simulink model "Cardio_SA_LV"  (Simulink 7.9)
settings: Solver=ode1  StartTime=0.0  StopTime=16*T  FixedStep=dt  MinStep=.001  RelTol=1e-3
PreLoadFcn:
  | %Time parameters
  | T = 0.0125;   %Duration of heartbeat (minutes)
  | Ts = 0.0050;   %Duration of systole   (minutes)
  | Stroke_volume = 70e-3;
  | Tmax = 0.0020;  %Time at which flow is max (minutes)
  | Qmax= Stroke_volume/(0.5*Ts);    %Max flow through aortic valve (liters/minute)
  | dt = .00005*T;
  | %This choice implies 20,000 timesteps per cardiac cycle
  | 
  | %Compliance and resistance parameters. Note that valve resistances are not
  | %supposed to be realistic, just small enough to be negligible
  | Csa = .00175; %Systemic arterial compliance (liters/(mmHg))
  | Rs = 17.86; %Systemic resistance (mmHg/(liters/minute))
  | Rmi = .01; %mitral valve resistance (mmHg/(liters/minute))
  | RAo = .01; %Aortic valve resistance (mmHg/(liters/minute))
  | 
  | Vlvd = .027; %Left ventricular volume when PLV = 0 (liters)
  | Vsad = .825; %Systemic arterial volume when Psa = 0 (liters)
  | Pla = 5; %Left atrial pressure (mmHg)
  | 
  | %Parameters for Clv(t)
  | CLVD = .0146; %Max (diastolic) value of CLV (liters/mmHg)
  | CLVS = .00003; %Min (systolic) value of CLV (liters/mmHg)
  | tauS = .0025; %CLV time constant during systole (minutes)
  | tauD = .001; %CLV time constant during diastole (minutes)
  | 
  | %Initialization parameters
  | Plvi = 5; %initial value of PLV (mmHg)
  | Psai = 80; %initial value of Psa (mmHg)
  | 
  | %Don't forget to plot VSA vs. PSA and VLV vs. PLV!!!!!!! The values have
  | %been exported into the matlab workspace so you can plot them yourself!

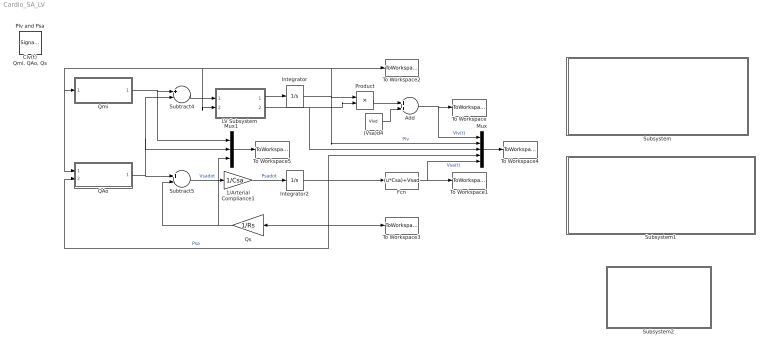
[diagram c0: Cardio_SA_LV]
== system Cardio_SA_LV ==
  (Vsa)d4 : Constant  Value=Vlvd
  1/Arterial Compliance1 : Gain  Gain=1/Csa
  Add : Sum
  Fcn : Fcn  Expr=(u*Csa)+Vsad
  Integrator : Integrator  InitialCondition=Plvi
  Integrator2 : Integrator  InitialCondition=Psai
  LV Subsystem : Subsystem
  Mux : Mux  Inputs=5
  Mux1 : Mux  Inputs=3
  Product : Product
  QAo : Subsystem
  Qmi : Subsystem
  Qs : Gain  Gain=1/Rs
  Subsystem : Subsystem
  Subsystem1 : Subsystem
  Subsystem2 : Subsystem
  Subtract4 : Sum  Inputs=+-
  Subtract5 : Sum  Inputs=+-
  To Workspace : ToWorkspace  VariableName=VLV  SampleTime=-1
  To Workspace1 : ToWorkspace  VariableName=VSA  SampleTime=-1
  To Workspace2 : ToWorkspace  VariableName=PLV  SampleTime=-1
  To Workspace3 : ToWorkspace  VariableName=PSA  SampleTime=-1
  To Workspace4 : ToWorkspace  VariableName=PVClv  SampleTime=-1  SaveFormat=Structure With Time
  To Workspace5 : ToWorkspace  VariableName=BloodFlows  SampleTime=-1  SaveFormat=Structure With Time
  Clv(t) : SignalViewerScope  IOType=viewer  RefreshTime=0.035000
  Plv and Psa : SignalViewerScope  IOType=viewer  RefreshTime=0.035000
  "Qmi, QAo, Qs" : SignalViewerScope  IOType=viewer  RefreshTime=0.035000
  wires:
  Fcn/1 -> To Workspace1/1, Mux/5  "Vsa(t)"
  Subtract5/1 -> 1/Arterial Compliance1/1  "Vsadot"
  1/Arterial Compliance1/1 -> Integrator2/1  "Psadot"
  Integrator2/1 -> Fcn/1, To Workspace3/1, Qs/1, QAo/2(Psa), Mux/4  "Psa"
  Qs/1 -> Subtract5/2, Mux1/3
  QAo/1(Qao) -> Subtract5/1, Subtract4/2, Mux1/2
  Qmi/1(Qmi) -> Subtract4/1, Mux1/1
  Product/1 -> Add/1
  (Vsa)d4/1 -> Add/2
  Add/1 -> To Workspace/1, Mux/1  "Vlv(t)"
  Subtract4/1 -> LV Subsystem/1(Vlddot)
  LV Subsystem/1(Plvdot) -> Integrator/1
  Integrator/1 -> Product/1, To Workspace2/1, LV Subsystem/2(Plv), Qmi/1(Plv), QAo/1(Plv), Mux/2  "Plv"
  LV Subsystem/2(Clv) -> Product/2, Mux/3
  Mux/1 -> To Workspace4/1
  Mux1/1 -> To Workspace5/1

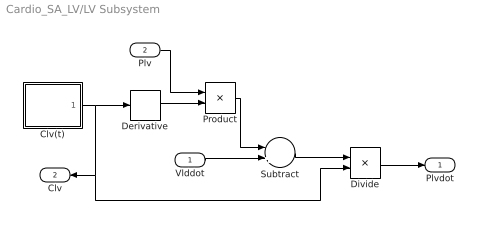
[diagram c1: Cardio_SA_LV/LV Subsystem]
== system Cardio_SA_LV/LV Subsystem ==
  Vlddot : Inport
  Plv : Inport  Port=2
  Clv(t) : Subsystem
  Derivative : Derivative
  Divide : Product  Inputs=*/
  Product : Product
  Subtract : Sum  Inputs=-+
  Plvdot : Outport
  Clv : Outport  Port=2
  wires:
  Clv(t)/1(Clv) -> Derivative/1, Clv/1, Divide/2
  Derivative/1 -> Product/2
  Plv/1 -> Product/1
  Product/1 -> Subtract/1
  Vlddot/1 -> Subtract/2
  Subtract/1 -> Divide/1
  Divide/1 -> Plvdot/1

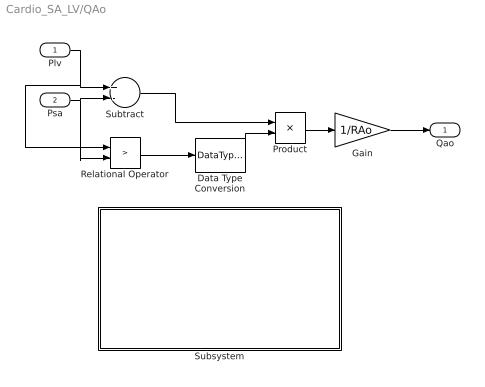
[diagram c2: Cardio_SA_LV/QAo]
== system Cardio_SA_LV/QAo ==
  Plv : Inport
  Psa : Inport  Port=2
  Data Type Conversion : DataTypeConversion  OutDataTypeStr=double
  Gain : Gain  Gain=1/RAo
  Product : Product
  Relational Operator : RelationalOperator  Operator=>  OutDataTypeStr=boolean
  Subsystem : Subsystem
  Subtract : Sum  Inputs=+-
  Qao : Outport
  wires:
  Plv/1 -> Subtract/1, Relational Operator/1
  Subtract/1 -> Product/1
  Product/1 -> Gain/1
  Gain/1 -> Qao/1
  Psa/1 -> Subtract/2, Relational Operator/2
  Data Type Conversion/1 -> Product/2
  Relational Operator/1 -> Data Type Conversion/1

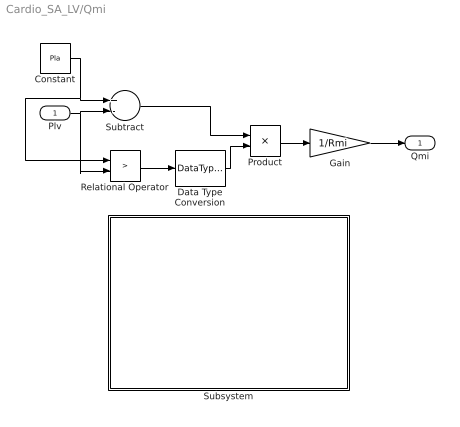
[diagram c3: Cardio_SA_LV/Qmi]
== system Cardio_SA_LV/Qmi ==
  Plv : Inport
  Constant : Constant  Value=Pla
  Data Type Conversion : DataTypeConversion  OutDataTypeStr=double
  Gain : Gain  Gain=1/Rmi
  Product : Product
  Relational Operator : RelationalOperator  Operator=>  OutDataTypeStr=boolean
  Subsystem : Subsystem
  Subtract : Sum  Inputs=+-
  Qmi : Outport
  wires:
  Constant/1 -> Relational Operator/1, Subtract/1
  Subtract/1 -> Product/1
  Product/1 -> Gain/1
  Gain/1 -> Qmi/1
  Plv/1 -> Relational Operator/2, Subtract/2
  Data Type Conversion/1 -> Product/2
  Relational Operator/1 -> Data Type Conversion/1

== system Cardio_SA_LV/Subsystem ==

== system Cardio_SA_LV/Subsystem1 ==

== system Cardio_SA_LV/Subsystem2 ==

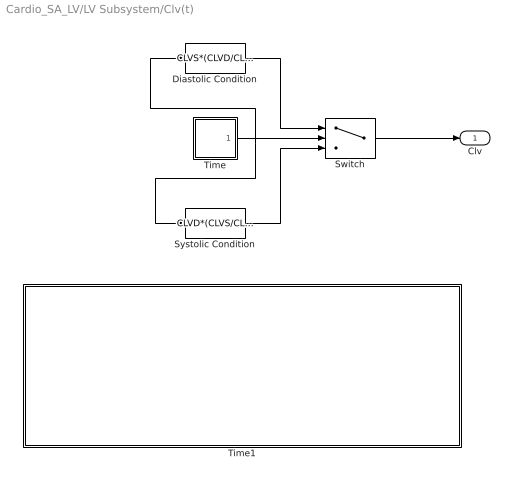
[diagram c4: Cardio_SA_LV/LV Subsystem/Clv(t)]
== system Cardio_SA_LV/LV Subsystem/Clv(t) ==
  Diastolic Condition : Fcn  Expr=CLVS*(CLVD/CLVS)^((1-exp(-(u-Ts)/tauD))/(1-exp(-(T-Ts)/tauD)))
  Switch : Switch  Criteria=u2 > Threshold  Threshold=Ts
  Systolic Condition : Fcn  Expr=CLVD*(CLVS/CLVD)^((1-exp(-u/tauS))/(1-exp(-Ts/tauS)))
  Time : Subsystem
  Time1 : Subsystem
  Clv : Outport
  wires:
  Time/1(Out1) -> Diastolic Condition/1, Systolic Condition/1, Switch/2
  Diastolic Condition/1 -> Switch/1
  Systolic Condition/1 -> Switch/3
  Switch/1 -> Clv/1

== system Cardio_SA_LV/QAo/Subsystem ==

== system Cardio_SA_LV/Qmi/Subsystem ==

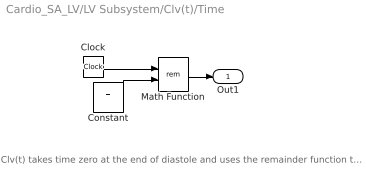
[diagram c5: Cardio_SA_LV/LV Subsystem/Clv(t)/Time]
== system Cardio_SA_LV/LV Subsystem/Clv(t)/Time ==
  note: Clv(t) takes time zero at the end of diastole and uses the remainder function to accomplish this
  Clock : Clock
  Constant : Constant  Value=T
  Math Function : Math  Operator=rem
  Out1 : Outport
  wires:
  Math Function/1 -> Out1/1
  Constant/1 -> Math Function/2
  Clock/1 -> Math Function/1

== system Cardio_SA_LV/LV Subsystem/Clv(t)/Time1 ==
